(* Logix 5000 AddOnInstructionDefinition export ACS_HOME_MOVE; software revision 20.01 *)

ADD_ON_INSTRUCTION ACS_HOME_MOVE   (* revision 2.0, vendor Tolomatic, Inc *)
// Initiated Homing Routine based on homing profile defined in drive
// Help:
// Add-On Instruction Executes Homing Routine
VAR_IN_OUT
   DriveCMD : SINT; {required}   // ACS.O.CMD
END_VAR

ROUTINE Logic   (* ladder *)
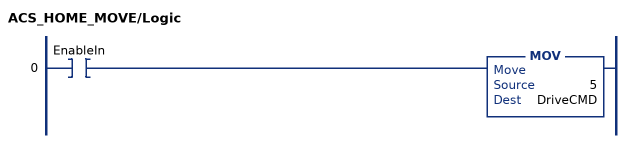
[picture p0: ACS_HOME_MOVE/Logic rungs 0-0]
   0: XIC(EnableIn)MOV(5,DriveCMD);
END_ROUTINE
END_ADD_ON_INSTRUCTION
